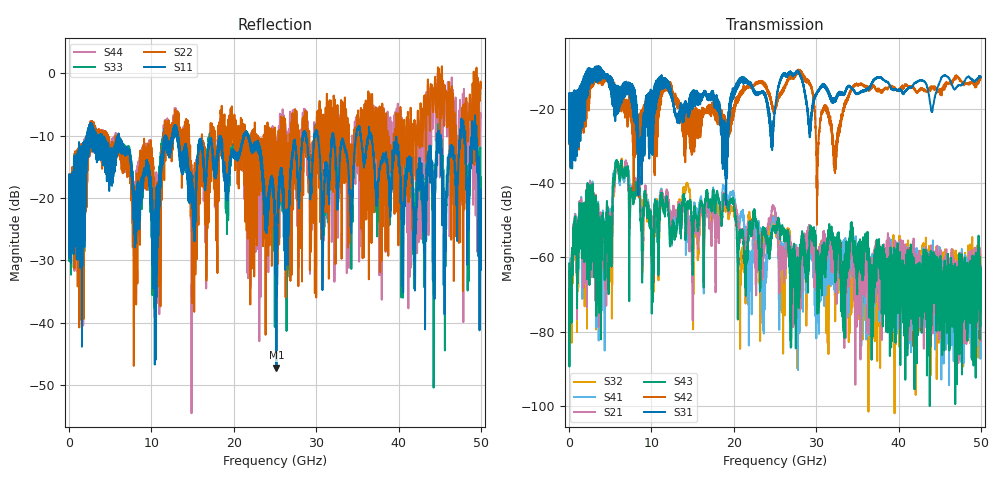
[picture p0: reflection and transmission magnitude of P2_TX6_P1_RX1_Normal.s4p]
!Keysight Technologies,N5225B,MY57041031,A.13.20.10
!Date: Friday, May 31, 2019 11:15:02
!Correction: S11(Full 4 Port(1,2,3,4))
!S12(Full 4 Port(1,2,3,4))
!S13(Full 4 Port(1,2,3,4))
!S14(Full 4 Port(1,2,3,4))
!S21(Full 4 Port(1,2,3,4))
!S22(Full 4 Port(1,2,3,4))
!S23(Full 4 Port(1,2,3,4))
!S24(Full 4 Port(1,2,3,4))
!S31(Full 4 Port(1,2,3,4))
!S32(Full 4 Port(1,2,3,4))
!S33(Full 4 Port(1,2,3,4))
!S34(Full 4 Port(1,2,3,4))
!S41(Full 4 Port(1,2,3,4))
!S42(Full 4 Port(1,2,3,4))
!S43(Full 4 Port(1,2,3,4))
!S44(Full 4 Port(1,2,3,4))
!S4P File: Measurements: <S11,S12,S13,S14>,
!<S21,S22,S23,S24>,
!<S31,S32,S33,S34>,
!<S41,S42,S43,S44>:
# Hz S  dB  R 50.0
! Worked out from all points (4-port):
!   5000 points, 10 MHz to 50 GHz, reference 50 ohm
!   strongest paths, dB at 10 MHz, 12.51 GHz, 25.01 GHz, 37.51 GHz, 50 GHz:
!     S31: -19.3, -16.8, -20.0, -11.7, -11.4
!     S42: -19.5, -14.6, -20.1, -14.8, -11.4
!     S43: -61.6, -53.7, -52.8, -60.8, -65.0
!     S21: -63.7, -51.6, -48.2, -56.9, -82.6
!     S41: -70.4, -51.1, -50.7, -65.7, -62.9
!     S32: -64.5, -50.8, -52.8, -65.6, -64.8
!   lowest |S11| = -47.2 dB at 25.18 GHz (marker M1), VSWR 1.01, Z = 50 - j0.435 ohm
!   |S11| at or under -10 dB: 13.21 GHz to 21.18 GHz (7.966 GHz wide, 46.3 % of centre); 21.74 GHz to 28.38 GHz (6.639 GHz wide, 26.5 % of centre); 36.67 GHz to 44.63 GHz (7.959 GHz wide, 19.6 % of centre)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
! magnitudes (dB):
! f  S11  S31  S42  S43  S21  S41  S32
! 10 MHz  -19.4  -19.3  -19.5  -61.6  -63.7  -70.4  -64.5
! 5.86 GHz  -11.9  -17.5  -15.9  -34.1  -34.5  -34.2  -34.3
! 10.11 GHz  -20.2  -15.5  -26.2  -56.5  -50.2  -54.3  -51.7
! 25.18 GHz  -47.2  -16.9  -19.0  -52.8  -51.3  -51.7  -54.6
! 28.57 GHz  -9.2  -15.0  -11.7  -59.2  -53.5  -63.4  -59.4
! 32.27 GHz  -12.0  -17.6  -32.2  -61.0  -59.1  -59.5  -70.3
! 50 GHz  -23.5  -11.4  -11.4  -65.0  -82.6  -62.9  -64.8
